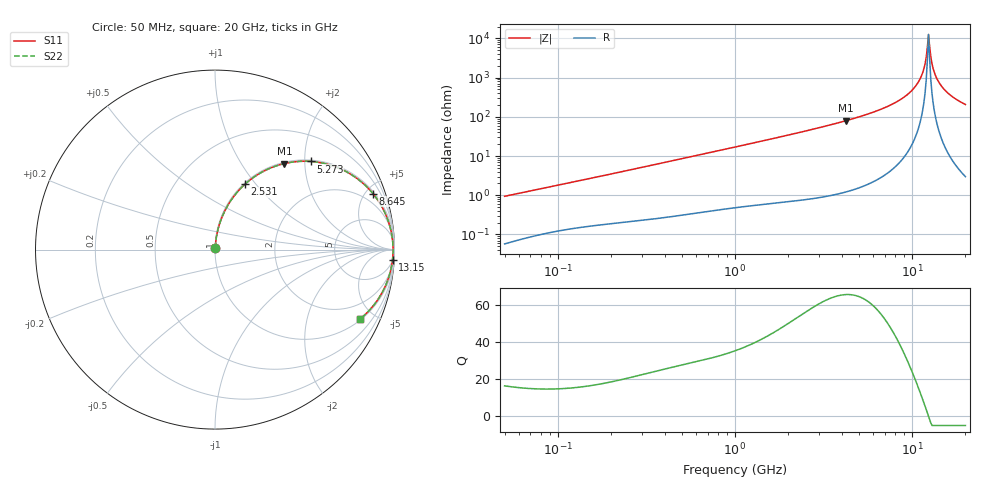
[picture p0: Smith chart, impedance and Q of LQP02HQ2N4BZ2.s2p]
!Murata Part Number: LQP02HQ2N4BZ2
!These Parameters are Measured in Series Mode Connection
!  o--[Z]--o
!Port1  Port2
!  o-------o
!Freq. Start=50[MHz] Stop=20[GHz], 401[Steps]
# Hz S RI R 50
!Freq.(Hz) S11(Real) S11(Imag) S21(Real) S21(Imag) S12(Real) S12(Imag) S22(Real) S22(Imag)
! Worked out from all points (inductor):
!   401 points, 50 MHz to 20 GHz, reference 50 ohm
!   read as one part in series: L = 2.95 nH near 51.52 MHz
!   highest Q = 65.6 at 4.212 GHz (marker M1), where L = 2.99 nH
!   self-resonance near 12.38 GHz
!   S11 on the Smith chart (normalised r, x): 50 MHz: 1.00, +0.02; 2.531 GHz: 1.02, +0.88; 5.273 GHz: 1.03, +2.14; 8.645 GHz: 1.15, +5.59; 13.15 GHz: 6, -34; 20 GHz: 1.06, -4.13
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5e7  0.000661 0.00937  0.9993 -0.00937  0.9993 -0.00937  0.000661 0.00937
1.364002e8  0.00211 0.0241  0.9979 -0.0241  0.9979 -0.0241  0.00211 0.0241
3.721004e8  0.00661 0.0633  0.9934 -0.0633  0.9934 -0.0633  0.00661 0.0633
1e9  0.0323 0.1632  0.9677 -0.1632  0.9677 -0.1632  0.0323 0.1632
2.531158e9  0.1665 0.3638  0.8335 -0.3638  0.8335 -0.3638  0.1665 0.3638
2.728004e9  0.1897 0.3836  0.8103 -0.3836  0.8103 -0.3836  0.1897 0.3836
4.212059e9  0.387 0.4795  0.613 -0.4795  0.613 -0.4795  0.387 0.4795
5.273168e9  0.5333 0.4911  0.4667 -0.4911  0.4667 -0.4911  0.5333 0.4911
7.442007e9  0.7843 0.4012  0.2157 -0.4012  0.2157 -0.4012  0.7843 0.4012
8.644534e9  0.8803 0.3115  0.1197 -0.3115  0.1197 -0.3115  0.8803 0.3115
9.892087e9  0.9461 0.2067  0.0539 -0.2067  0.0539 -0.2067  0.9461 0.2067
1.098561e10  0.9786 0.1135  0.0214 -0.1135  0.0214 -0.1135  0.9786 0.1135
1.149051e10  0.9867 0.0714  0.0133 -0.0714  0.0133 -0.0714  0.9867 0.0714
1.183995e10  0.9901 0.043  0.00988 -0.043  0.00988 -0.043  0.9901 0.043
1.201863e10  0.9912 0.0287  0.0088 -0.0287  0.0088 -0.0287  0.9912 0.0287
1.238412e10  0.9921 9.19e-05  0.00787 -9.19e-05  0.00787 -9.19e-05  0.9921 9.19e-05
1.276073e10  0.9914 -0.0286  0.00861 0.0286  0.00861 0.0286  0.9914 -0.0286
1.314879e10  0.989 -0.0571  0.011 0.0571  0.011 0.0571  0.989 -0.0571
1.396067e10  0.9793 -0.1135  0.0207 0.1135  0.0207 0.1135  0.9793 -0.1135
1.504638e10  0.9583 -0.1812  0.0417 0.1812  0.0417 0.1812  0.9583 -0.1812
1.696185e10  0.9065 -0.2798  0.0935 0.2798  0.0935 0.2798  0.9065 -0.2798
2e10  0.8066 -0.3878  0.1934 0.3878  0.1934 0.3878  0.8066 -0.3878
